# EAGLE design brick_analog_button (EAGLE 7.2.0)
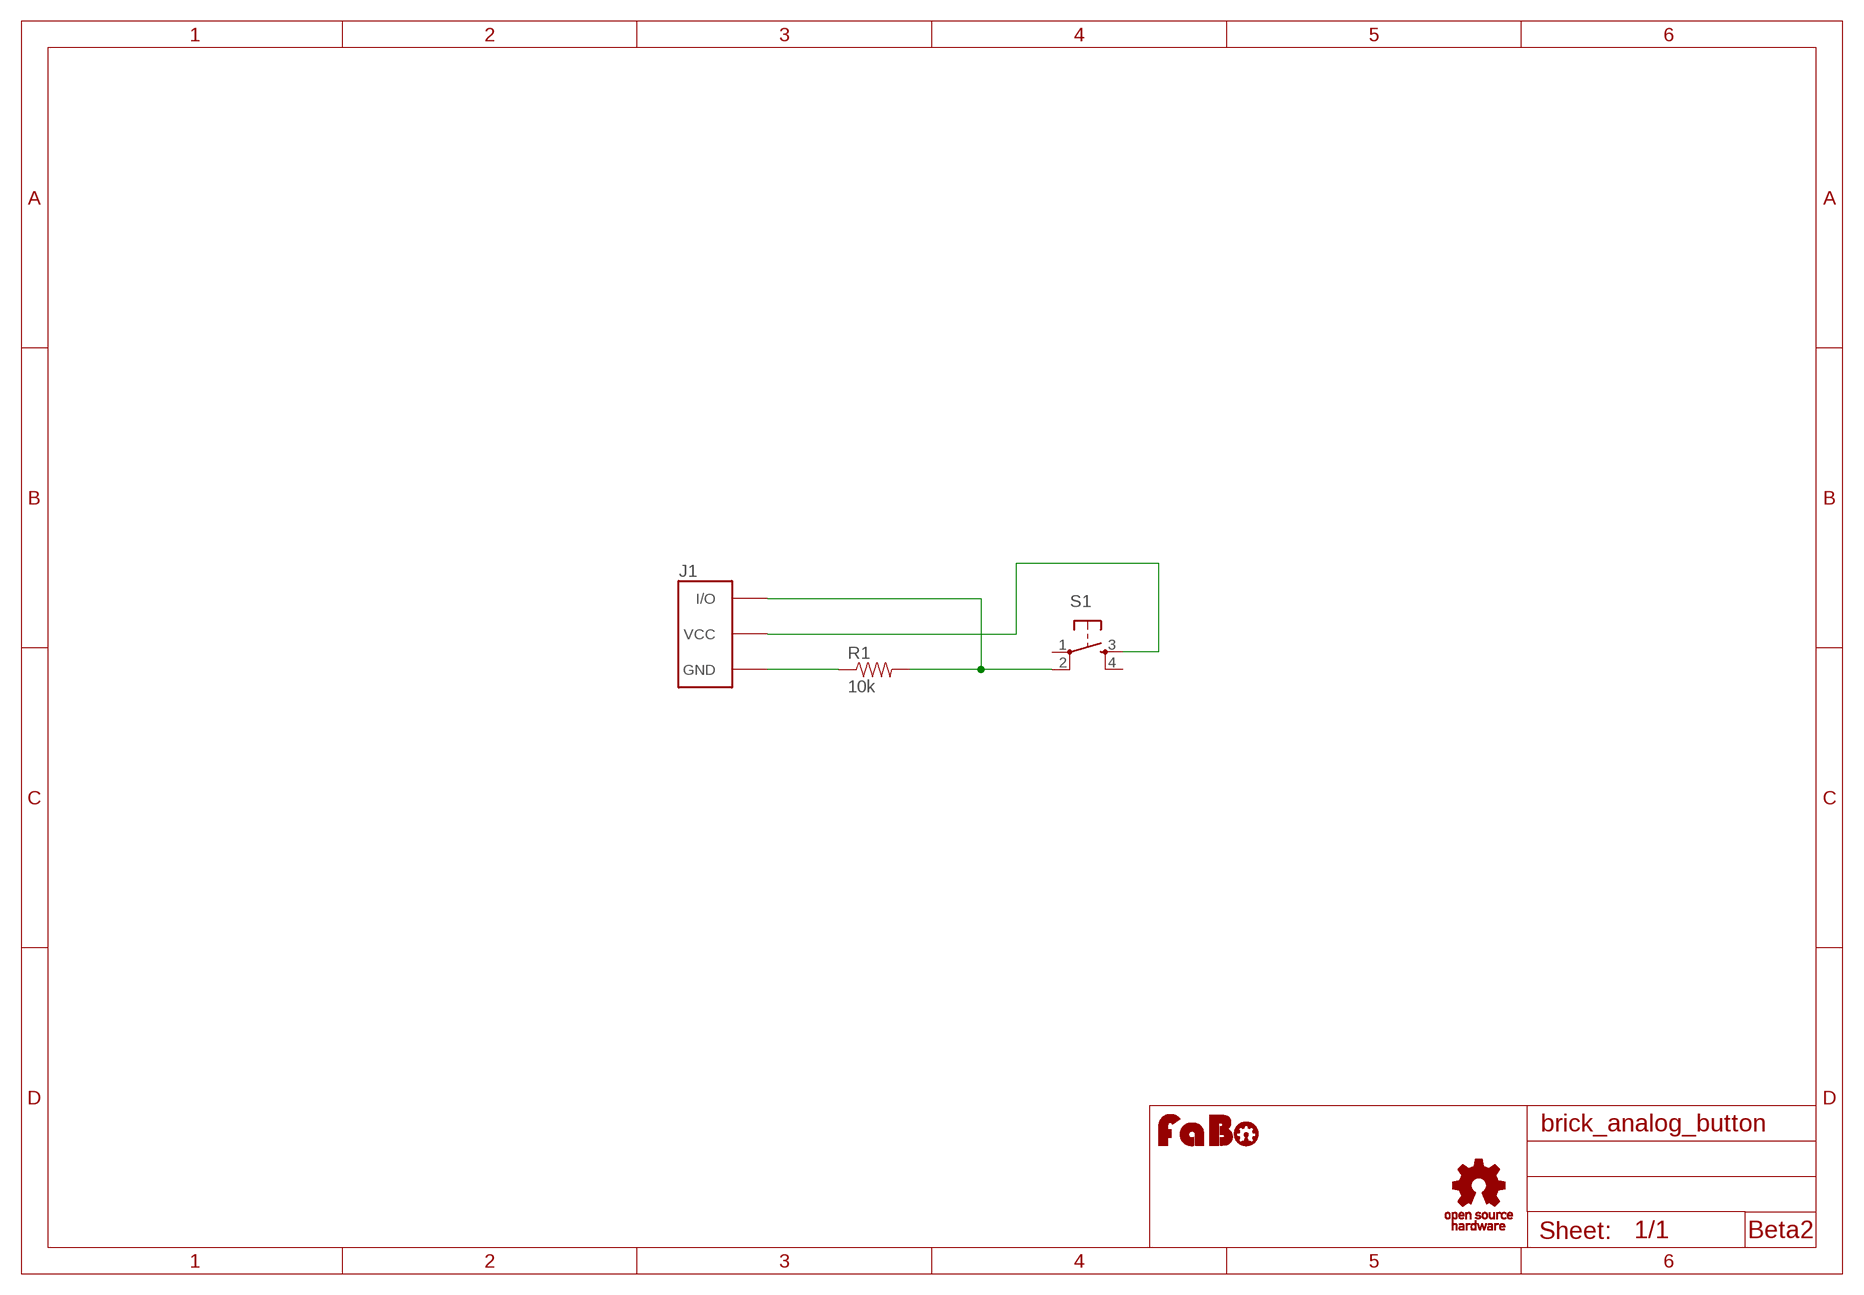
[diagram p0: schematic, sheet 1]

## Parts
J1  BRICK_3PIN  [BRICK_3PIN]
R1  10k  RES-PTH-REGULAR  [RES-AXL-REGULAR]
S1  SWITCH-TACT-6MM  [DTS_6_V]
U$2  LOGO_FABO-M  [LOGO_FABO_M]
U$3  LOGO_OSHW_T-M  [LOGO_OSHW_T_M]

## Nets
GND: J1.GND R1.P$1
N$1: J1.VCC S1.3
N$4: J1.IN/OUT(I/O) R1.P$2 S1.2
Unconnected: S1.1 S1.4

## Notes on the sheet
- Beta2

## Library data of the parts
J1 = gclue:BRICK_3PIN: FaBo Brick 3pin
R1 = gclue:RES
S1 = gclue:SWITCH-TACT
U$2 = FaBo:LOGO_FABO
U$3 = gclue:LOGO_OSHW_T

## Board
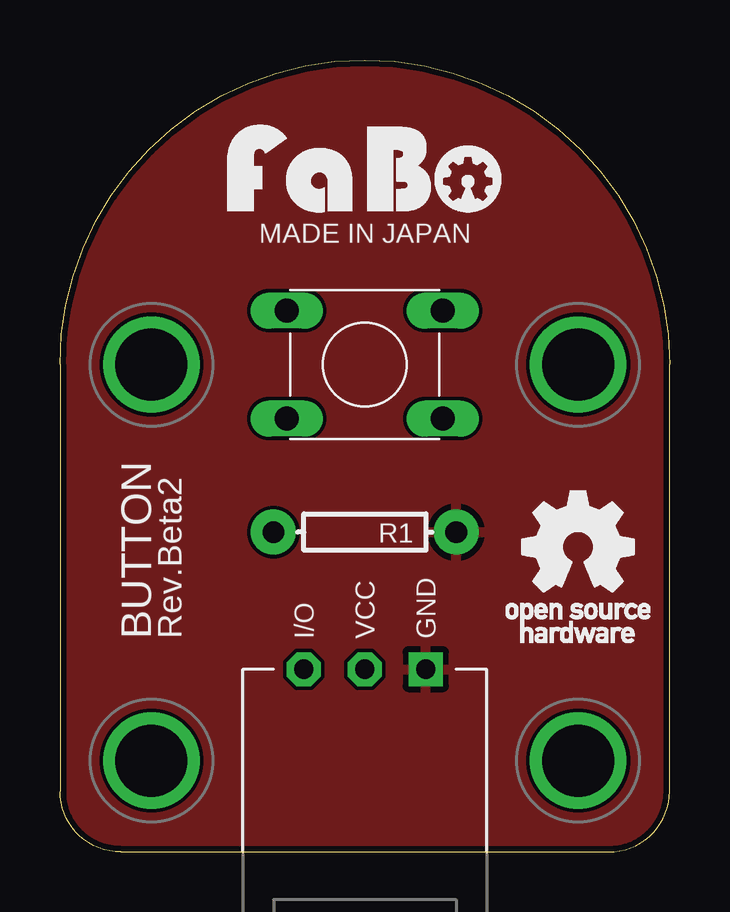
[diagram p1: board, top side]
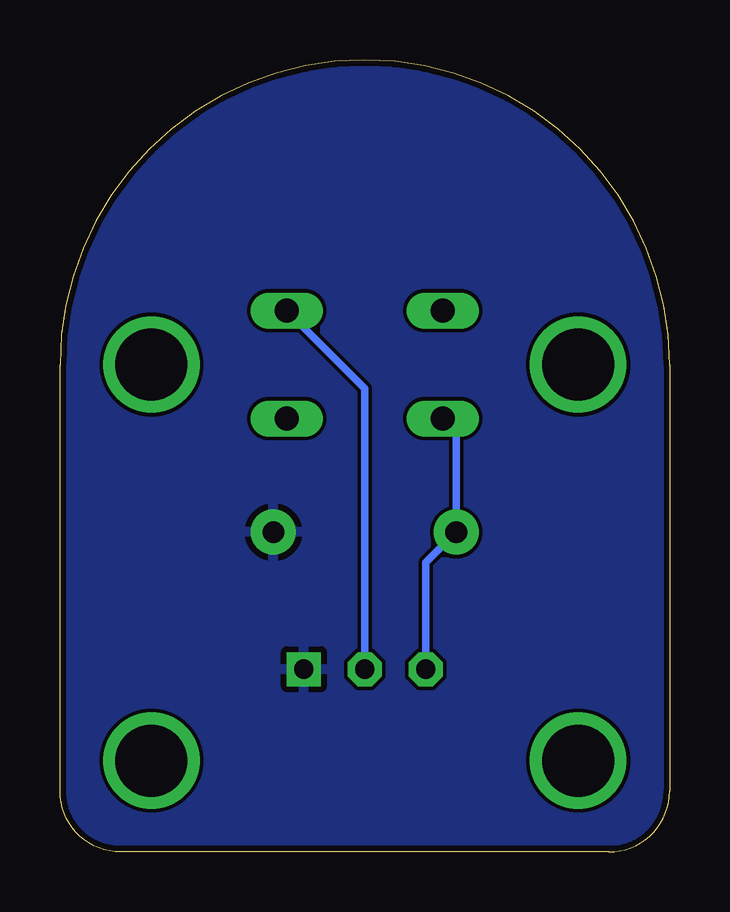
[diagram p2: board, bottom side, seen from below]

Size 25.4 x 33.02 mm. Coordinates in mm from the lower left corner, seen from the top.
Copper layers (1*16): Top 0.035mm / dielectric 1.5mm / Bottom 0.035mm
Design rules "Elecrow_2-layer_eagle_rule": minimum track width 6mil, minimum drill 12mil, track to track 6mil, track to pad 6mil, pad to pad 6mil, via to via 6mil, smd to smd 0mil, copper to edge 10mil, drill to drill 10mil, minimum pad ring 10mil, minimum via ring 6mil, stop-mask expansion 2mil, vias tented up to drill 100mil, thermal gap 10mil

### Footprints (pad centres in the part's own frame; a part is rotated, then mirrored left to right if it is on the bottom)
BRICK_3PIN = drill 0.8 pad 1.422 square: GND 2.54,-8.89 | drill 0.8 pad 1.422 octagon: IN/OUT -2.54,-8.89; VCC 0,-8.89 | drill 3 pad 3.81: P$5 -8.89,3.81; P$6 8.89,3.81; P$7 -8.89,-12.7; P$8 8.89,-12.7
RES-AXL-REGULAR = drill 0.9 pad 1.88: P$1 -3.81,0; P$2 3.81,0
DTS_6_V = drill 1 long: 1 -3.25,2.25; 2 3.25,2.25; 3 -3.25,-2.25; 4 3.25,-2.25

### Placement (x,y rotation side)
J1  12.7,16.51 0 top
R1  12.7,13.34 180 top
S1  12.7,20.32 180 top
U$2  12.7,26.67 0 top
U$3  21.59,12.7 0 top

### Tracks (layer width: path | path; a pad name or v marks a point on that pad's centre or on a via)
GND
  pour Bottom: -1.27,-1.27 26.67,-1.27 26.67,34.29 -1.27,34.29
  pour Top: -1.27,-1.27 26.67,-1.27 26.67,34.29 -1.27,34.29
N$1
  Bottom 0.305: J1.VCC 12.7,19.32 S1.3
N$4
  Bottom 0.305: S1.2 8.89,17.51 R1.P$2 10.16,12.06 J1.IN/OUT

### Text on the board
tPlace: MADE IN JAPAN | BUTTON | Rev.Beta2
